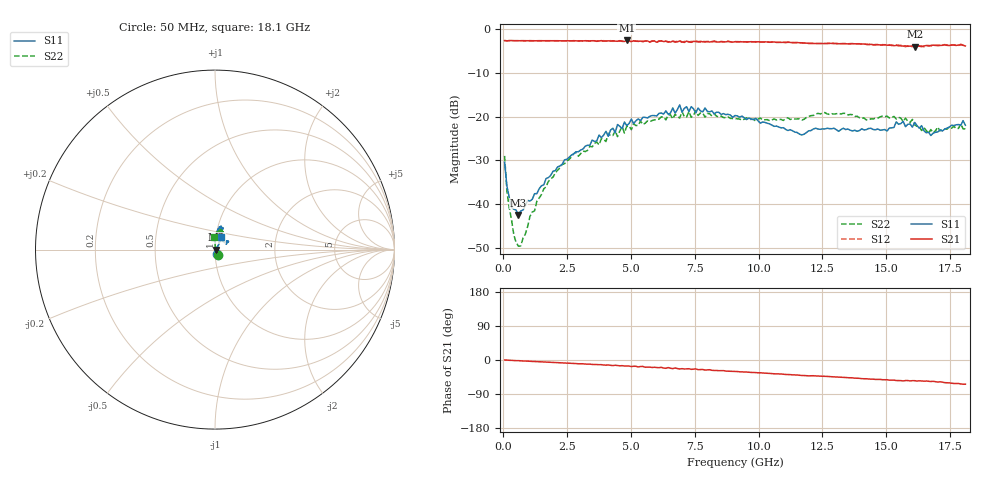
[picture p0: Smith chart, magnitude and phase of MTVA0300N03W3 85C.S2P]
! Network Analyzer HP8720D.06.14 Serial No. US36140669
!  7 Jul 2005  08:36:24
! Frequency  S11  S21  S12  S22
# HZ  S  DB R 50
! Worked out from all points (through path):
!   201 points, 50 MHz to 18.1 GHz, reference 50 ohm
!   highest |S21| = -2.56 dB at 4.833 GHz (marker M1); lowest = -4.0 dB at 16.11 GHz (marker M2)
!   group delay of S21, straight-line fit = 9.71 ps
!   lowest |S11| = -42.6 dB at 591.5 MHz (marker M3), VSWR 1.02, Z = 50.7 + j0.0401 ohm
!   |S11| at or under -10 dB: start of sweep to end of sweep
!   |S22| runs from -49.7 to -18.7 dB; largest |S21 - S12| = 0.027
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5e7  -30.49 -65.7  -2.60 0.1  -2.59 0.2  -29.01 -61.3
1.4025e8  -35.93 -53.1  -2.64 -0.4  -2.64 -0.3  -37.13 -66.3
2.305e8  -38.48 -39.6  -2.61 -0.7  -2.60 -0.7  -40.81 -62.2
4.11e8  -41.22 -21.3  -2.63 -1.4  -2.62 -1.4  -47.11 -37.5
5.915e8  -42.55 3.0  -2.60 -1.7  -2.63 -1.8  -49.69 18.0
1.76475e9  -33.97 50.7  -2.62 -5.8  -2.62 -5.8  -34.85 84.6
3.1185e9  -27.44 60.0  -2.65 -9.9  -2.68 -10.3  -27.88 92.7
4.021e9  -23.38 64.2  -2.68 -13.5  -2.70 -13.0  -25.72 87.0
4.11125e9  -24.51 64.0  -2.66 -12.9  -2.69 -13.8  -23.84 86.8
4.47225e9  -21.81 61.3  -2.75 -14.7  -2.65 -14.2  -24.59 90.6
4.83325e9  -22.07 71.0  -2.56 -15.7  -2.68 -16.3  -22.25 79.2
6.09675e9  -19.27 70.0  -2.75 -20.3  -2.66 -20.2  -20.59 77.1
6.7285e9  -19.20 77.1  -2.83 -21.0  -2.99 -21.8  -19.46 70.5
6.909e9  -17.33 75.8  -2.64 -23.7  -2.74 -22.6  -20.34 69.9
7.54075e9  -19.14 72.6  -2.83 -23.6  -2.69 -25.5  -18.65 75.3
9.075e9  -19.76 82.3  -2.85 -30.1  -2.83 -30.2  -20.45 66.2
1.169225e10  -24.20 73.4  -3.13 -40.9  -3.13 -40.8  -20.79 74.9
1.21435e10  -22.84 70.7  -3.26 -41.5  -3.21 -41.6  -19.74 77.9
1.512175e10  -22.61 31.9  -3.66 -53.2  -3.53 -52.8  -20.30 80.8
1.61145e10  -21.33 31.2  -4.00 -54.6  -3.75 -55.1  -21.90 71.3
1.674625e10  -24.34 47.6  -3.70 -56.7  -3.81 -57.1  -22.97 85.1
1.81e10  -21.99 64.8  -3.83 -63.8  -3.90 -64.9  -22.80 94.5
